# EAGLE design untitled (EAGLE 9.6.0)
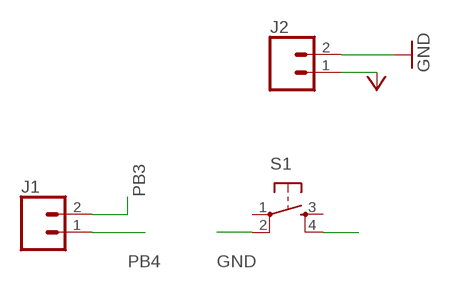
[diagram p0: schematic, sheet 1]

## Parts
J1  CONN_02  [1X02]
J2  CONN_02  [1X02]
S1  SW_SWITCH_TACTILE_6MM6MM_SWITCH  [6MM_SWITCH]

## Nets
GND: J2.2 S1.2(P1)
PB3: J1.2
PB4: J1.1 S1.4(S1)
VCC: J2.1
Unconnected: S1.1(P) S1.3(S)

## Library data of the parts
J1 J2 = SparkFun-Connectors:CONN_02: Multi connection point. Often used as Generic Header-pin footprint for 0.1 inch spaced/style header connections
S1 = fab:SW_SWITCH_TACTILE_6MM: OMRON SWITCH

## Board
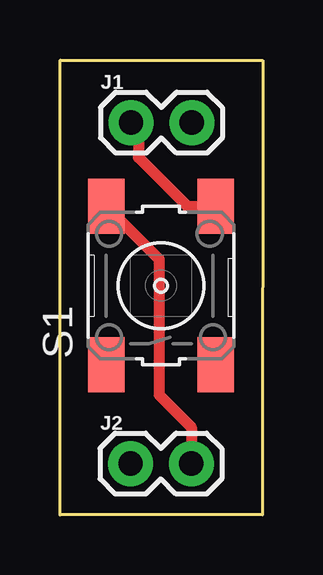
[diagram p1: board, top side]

Size 8.46 x 18.95 mm. Coordinates in mm from the lower left corner, seen from the top.
Outline: 0.01,18.95 8.46,18.93 8.45,0 0,0 0.01,18.95
Copper layers (1*16): Top 0.035mm / dielectric 1.5mm / Bottom 0.035mm
Design rules "default *": minimum track width 18mil, minimum drill 0.35mm, track to track 16mil, track to pad 16mil, pad to pad 16mil, via to via 6mil, smd to smd 16mil, copper to edge 40mil, drill to drill 6mil, minimum pad ring 10mil, minimum via ring 8mil, stop-mask expansion 4mil, vias tented up to drill 0mil, thermal gap 10mil

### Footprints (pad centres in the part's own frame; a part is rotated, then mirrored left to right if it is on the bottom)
1X02 = drill 1.016 pad 1.88: 1 0,0; 2 2.54,0
6MM_SWITCH = smd 2.286 x 1.524: 1 -3.302,2.286; 2 3.302,2.286; 3 -3.302,-2.286; 4 3.302,-2.286

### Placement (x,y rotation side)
J1  2.97,16.34 0 top
J2  2.95,2.13 0 top
S1  4.22,9.55 90 top

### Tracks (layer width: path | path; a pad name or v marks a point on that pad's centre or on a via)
GND
  Top 0.457: S1.2 4.14,10.65 4.14,5 5.49,3.65 J2.2
PB4
  Top 0.457: J1.1 3.28,16.03 3.28,14.89 5.31,12.85 S1.4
